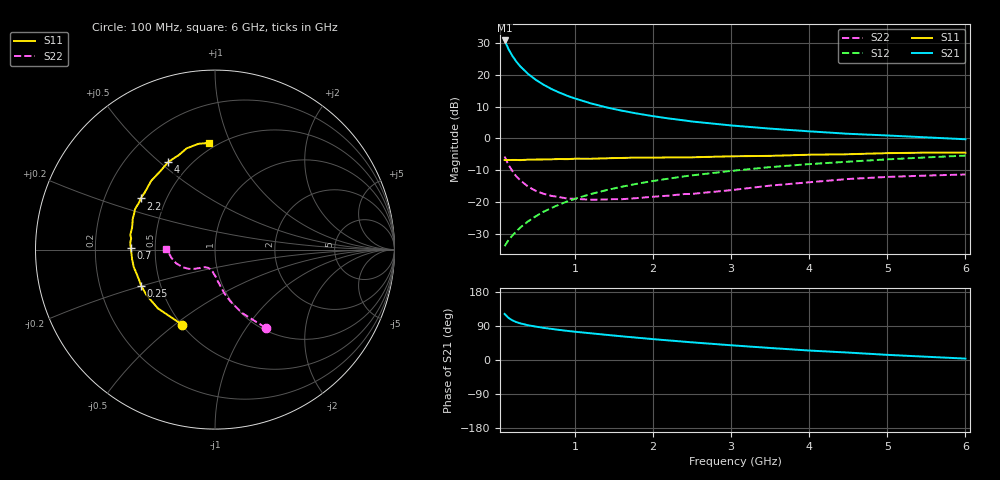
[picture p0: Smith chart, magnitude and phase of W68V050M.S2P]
! SIEMENS Small Signal Semiconductors
! BFR193W
! Si NPN RF Bipolar Junction Transistor in SOT323
! VCE = 8 V  IC = 50 mA
! Common Emitter S-Parameters:  September  1992
# GHz  S  MA  R  50
!  f  S11  S21  S12  S22
! GHz  MAG  ANG  MAG  ANG  MAG  ANG  MAG  ANG
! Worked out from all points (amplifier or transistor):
!   28 points, 100 MHz to 6 GHz, reference 50 ohm
!   highest |S21| = 30.8 dB at 100 MHz (marker M1)
!   |S21| within 3 dB of that: start of sweep to 156.5 MHz
!   unconditionally stable (mu >= 1): 578.8 MHz to 2.637 GHz
!   at 300 MHz: K = 0.90, MSG = 25.4 dB, |S12| = -28.0 dB
!   at 1.5 GHz: K = 1.03, MAG = 11.4 dB, |S12| = -15.7 dB
!   at 6 GHz: K = 0.92, MSG = 2.6 dB, |S12| = -5.4 dB
!   S11 on the Smith chart (normalised r, x): 100 MHz: 0.50, -0.53; 250 MHz: 0.39, -0.20; 700 MHz: 0.36, +0.01; 2.2 GHz: 0.36, +0.27; 4 GHz: 0.38, +0.54; 6 GHz: 0.45, +0.84
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0.1  0.457 -113.6  34.64 121.6  0.0202 60.1  0.5184 -57.1
0.15  0.4565 -134.2  25.33 111.1  0.0253 60.9  0.3838 -66.9
0.2  0.4581 -146.1  19.77 104.5  0.0297 62.5  0.3057 -73.0
0.25  0.4581 -154.0  16.12 100.1  0.0347 64.7  0.2524 -77.7
0.3  0.4554 -159.4  13.6 96.7  0.0396 66.2  0.2197 -80.3
0.4  0.4629 -167.9  10.32 91.8  0.0495 68.8  0.1748 -85.2
0.5  0.465 -173.2  8.317 88.1  0.0598 70.4  0.1493 -88.9
0.6  0.4662 -177.7  6.966 84.9  0.0704 71.1  0.1346 -93.0
0.7  0.469 179.0  5.973 82.0  0.0806 71.6  0.1247 -95.8
0.8  0.4739 175.4  5.258 79.4  0.0911 71.6  0.1194 -99.0
0.9  0.4713 172.5  4.681 76.9  0.1018 71.7  0.1135 -101.2
1  0.4789 170.0  4.247 74.6  0.1122 71.3  0.1121 -103.6
1.2  0.4779 165.1  3.564 70.5  0.1331 70.4  0.1085 -109.5
1.4  0.4864 160.7  3.081 66.5  0.1533 69.3  0.1095 -113.5
1.6  0.4921 156.6  2.729 62.5  0.1738 68.0  0.1105 -117.8
2.2  0.5021 145.4  2.058 51.7  0.2331 63.5  0.1259 -126.4
3  0.5227 132.9  1.597 38.9  0.3079 56.9  0.1535 -135.9
3.5  0.531 125.7  1.424 31.7  0.3534 52.6  0.181 -143.6
4  0.5534 118.0  1.291 25.0  0.394 48.1  0.2042 -151.2
4.5  0.5634 111.1  1.181 19.6  0.4303 44.0  0.2299 -160.7
5.5  0.5965 98.9  1.038 8.6  0.5023 35.9  0.2602 -176.7
6  0.5957 93.1  0.969 3.7  0.5362 31.8  0.2705 179.2
